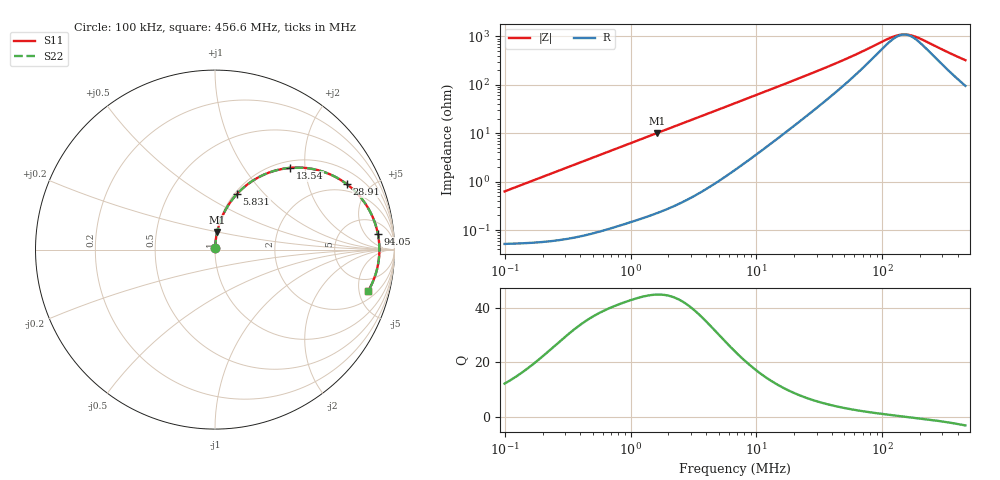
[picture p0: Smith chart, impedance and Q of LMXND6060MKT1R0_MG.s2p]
! LMXND6060MKT1R0_MG  S-PARAMETER MODEL  ( General Type )
! Model Generated by TAIYO YUDEN Corporation (http://www.ty-top.com)
! Version 1.0
! TAIYO YUDEN Control No. 191025NI43SB-FBB
! Copyright(c) 2019 TAIYO YUDEN CO.,LTD. All Rights Reserved.
! Product Description (link to TY-COMPAS)
! https://ds.yuden.co.jp/TYCOMPAS/or/detail?pn=LMXND6060MKT1R0NMG&u=M
! Products Name : Inductors
! Characteristics :
!  Inductance : 1.0 uH , SRF(min) : 95 MHz , DC Resistance(max) : 0.06 Ohm
!  Rated Current : Saturation :3000 mA , Temp Rise : 2400 mA
!  Case Size : 6.0 x 6.0 / 0.236 x 0.236 [mm/inch] , Thickness : 1.2 / 0.047 [mm/inch]
!  (Conditions: Temperature = 25 degC , DC Bias Current/Voltage = 0A / 0V)
! External Node Assignments :
!  1  o---GGG---o  2
! GND o---------o GND
! Frequency Range : 0.1MHz  -  456.598367MHz  [ 402 STEP ]
# MHz S RI R 50
! Freq[MHz].  S11 Real  S11 Imag  S21 Real  S21 Imag  S12 Real  S12 Imag  S22 Real  S22 Imag
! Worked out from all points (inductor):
!   401 points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, 100 kHz to 456.6 MHz, reference 50 ohm
!   read as one part in series: L = 996 nH near 104.3 kHz
!   highest Q = 44.7 at 1.613 MHz (marker M1), where L = 982 nH
!   self-resonance near 149.4 MHz
!   S11 on the Smith chart (normalised r, x): 100 kHz: 1.00, +0.01; 5.831 MHz: 1.03, +0.72; 13.54 MHz: 1.13, +1.67; 28.91 MHz: 1.61, +3.59; 94.05 MHz: 10, +11; 456.6 MHz: 2.89, -6.14
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0.1  0.000556 0.00625  0.9994 -0.00625  0.9994 -0.00625  0.000556 0.00625
0.410178  0.0014 0.0255  0.9986 -0.0255  0.9986 -0.0255  0.0014 0.0255
0.875649  0.00423 0.054  0.9958 -0.054  0.9958 -0.054  0.00423 0.054
1.613044  0.012 0.0981  0.988 -0.0981  0.988 -0.0981  0.012 0.0981
1.682457  0.0129 0.1022  0.9871 -0.1022  0.9871 -0.1022  0.0129 0.1022
3.443534  0.0478 0.2005  0.9522 -0.2005  0.9522 -0.2005  0.0478 0.2005
5.830762  0.1229 0.3102  0.8771 -0.3102  0.8771 -0.3102  0.1229 0.3102
6.901063  0.163 0.3487  0.837 -0.3487  0.837 -0.3487  0.163 0.3487
9.465609  0.2651 0.4142  0.7349 -0.4142  0.7349 -0.4142  0.2651 0.4142
13.54187  0.4179 0.4554  0.5821 -0.4554  0.5821 -0.4554  0.4179 0.4554
18.96969  0.573 0.4427  0.427 -0.4427  0.427 -0.4427  0.573 0.4427
27.71655  0.7211 0.3744  0.2789 -0.3744  0.2789 -0.3744  0.7211 0.3744
28.90925  0.7346 0.3646  0.2654 -0.3646  0.2654 -0.3646  0.7346 0.3646
48.95057  0.8528 0.2319  0.1472 -0.2319  0.1472 -0.2319  0.8528 0.2319
94.05279  0.9076 0.0869  0.0924 -0.0869  0.0924 -0.0869  0.9076 0.0869
113.6871  0.9132 0.0504  0.0868 -0.0504  0.0868 -0.0504  0.9132 0.0504
129.0043  0.9152 0.0269  0.0848 -0.0269  0.0848 -0.0269  0.9152 0.0269
143.3337  0.9159 0.00756  0.0841 -0.00756  0.0841 -0.00756  0.9159 0.00756
173.2558  0.9152 -0.0272  0.0848 0.0272  0.0848 0.0272  0.9152 -0.0272
205.0589  0.9122 -0.0587  0.0878 0.0587  0.0878 0.0587  0.9122 -0.0587
293.3653  0.8971 -0.1302  0.1029 0.1302  0.1029 0.1302  0.8971 -0.1302
456.5984  0.8527 -0.2323  0.1473 0.2323  0.1473 0.2323  0.8527 -0.2323
